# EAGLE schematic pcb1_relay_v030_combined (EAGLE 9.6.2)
Minor corrections.

## Sheet 1 of 3: Signal Generator
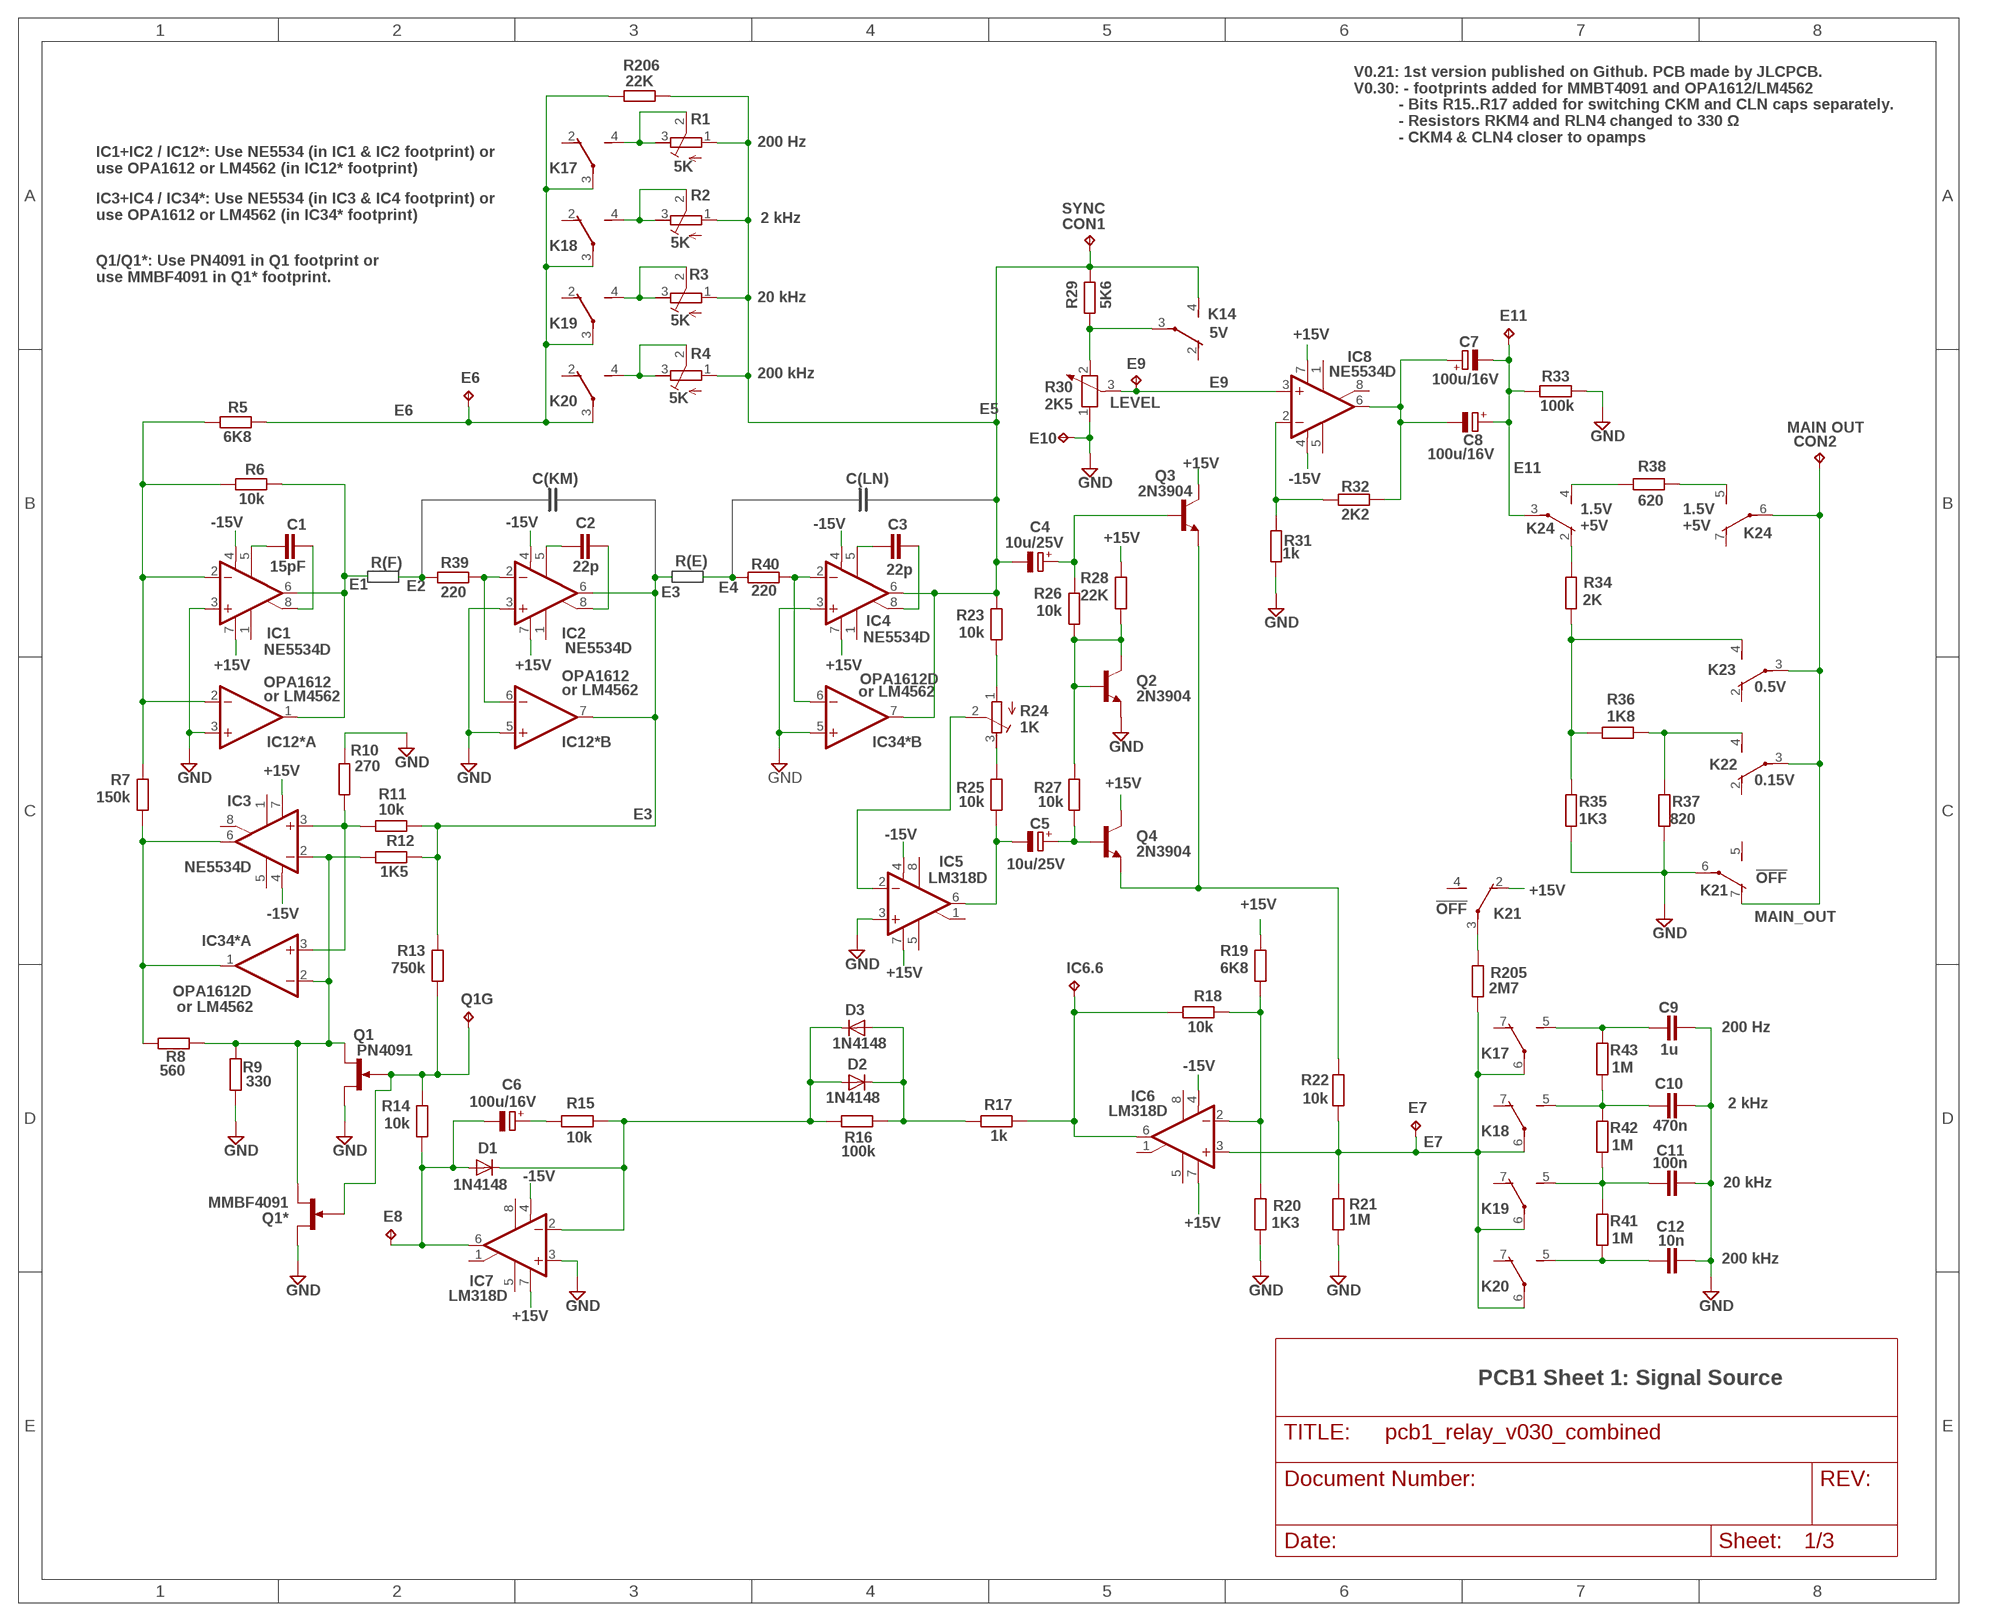
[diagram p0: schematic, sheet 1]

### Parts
C1  15pF  C-EU075-042X103  [C075-042X103]
C2  22p  C-EU075-042X103  [C075-042X103]
C3  22p  C-EU075-042X103  [C075-042X103]
C4  10u/25V  CPOL-EUUD-4X5,8  [UD-4X5,8_NICHICON]
C5  10u/25V  CPOL-EUUD-4X5,8  [UD-4X5,8_NICHICON]
C6  100u/16V  CPOL-EUUD-6,3X8,8  [UD-6,3X5,8_NICHICON]
C7  100u/16V  CPOL-EUUD-6,3X8,8  [UD-6,3X5,8_NICHICON]
C8  100u/16V  CPOL-EUUD-6,3X8,8  [UD-6,3X5,8_NICHICON]
C9  1u  C-EU150-072X183  [C150-072X183]
C10  470n  C-EU102-064X133  [C102-064X133]
C11  100n  C-EU075-063X106  [C075-063X106]
C12  10n  C-EU050-045X075  [C050-045X075]
CON1  MAIN_OUT  TPPAD1-13Y  [P1-13Y]
CON2  MAIN_OUT  TPPAD1-13Y  [P1-13Y]
D1  1N4148  D-SOD-80  [SOD80]
D2  1N4148  D-SOD-80  [SOD80]
D3  1N4148  D-SOD-80  [SOD80]
E6  TPPAD1-13Y  [P1-13Y]
E7  TPPAD1-13Y  [P1-13Y]
E8  TPPAD1-13Y  [P1-13Y]
E9  TPPAD1-13Y  [P1-13Y]
E10  MAIN_OUT  TPPAD1-13Y  [P1-13Y]
E11  TPPAD1-13Y  [P1-13Y]
IC1  NE5534D  NE5534AD  [SO08]
IC2  NE5534D  NE5534AD  [SO08]
IC3  NE5534D  NE5534AD  [SO08]
IC4  NE5534D  NE5534AD  [SO08]
IC5  LM318D  [SO08]
IC6  LM318D  [SO08]
IC6.6  TPPAD1-13Y  [P1-13Y]
IC7  LM318D  [SO08]
IC8  NE5534D  NE5534AD  [SO08]
IC12*  OPA1612  OPA1013D  [SO08]
IC34*  OPA1612D  OPA1013D  [SO08]
K14  G6K-2F-Y  [G6K-2F-Y]
K17  G6K-2F-Y  [G6K-2F-Y]
K18  G6K-2F-Y  [G6K-2F-Y]
K19  G6K-2F-Y  [G6K-2F-Y]
K20  G6K-2F-Y  [G6K-2F-Y]
K21  G6K-2F-Y  [G6K-2F-Y]
K22  G6K-2F-Y  [G6K-2F-Y]
K23  G6K-2F-Y  [G6K-2F-Y]
K24  G6K-2F-Y  [G6K-2F-Y]
Q1  PN4091  2N5638  [TO92G]
Q1*  MMBF4091  MMBFJ3  [SOT23]
Q1G  TPPAD1-13Y  [P1-13Y]
Q2  2N3904  [TO92]
Q3  2N3904  [TO92]
Q4  2N3904  [TO92]
R1  5K  R-TRIMM3296W  [RTRIM3296W]
R2  5K  R-TRIMM3296W  [RTRIM3296W]
R3  5K  R-TRIMM3296W  [RTRIM3296W]
R4  5K  R-TRIMM3296W  [RTRIM3296W]
R5  6K8  R-EU_R1206  [R1206]
R6  10k  R-EU_R1206  [R1206]
R7  150k  R-EU_R1206  [R1206]
R8  560  R-EU_R1206  [R1206]
R9  330  R-EU_R1206  [R1206]
R10  270  R-EU_R1206  [R1206]
R11  10k  R-EU_R1206  [R1206]
R12  1K5  R-EU_R1206  [R1206]
R13  750k  R-EU_R1206  [R1206]
R14  10k  R-EU_R1206  [R1206]
R15  10k  R-EU_R1206  [R1206]
R16  100k  R-EU_R1206  [R1206]
R17  1k  R-EU_R1206  [R1206]
R18  10k  R-EU_R1206  [R1206]
R19  6K8  R-EU_R1206  [R1206]
R20  1K3  R-EU_R1206  [R1206]
R21  1M  R-EU_R1206  [R1206]
R22  10k  R-EU_R1206  [R1206]
R23  10k  R-EU_R1206  [R1206]
R24  1K  R-TRIMM3296W  [RTRIM3296W]
R25  10k  R-EU_R1206  [R1206]
R26  10k  R-EU_R1206  [R1206]
R27  10k  R-EU_R1206  [R1206]
R28  22K  R-EU_R1206  [R1206]
R29  5K6  R-EU_R1206  [R1206]
R30  2K5  POTENTIOMETER_PT-10S  [PT-10S]
R31  1k  R-EU_R1206  [R1206]
R32  2K2  R-EU_R1206  [R1206]
R33  100k  R-EU_R1206  [R1206]
R34  2K  R-EU_R1206  [R1206]
R35  1K3  R-EU_R1206  [R1206]
R36  1K8  R-EU_R1206  [R1206]
R37  820  R-EU_R1206  [R1206]
R38  620  R-EU_R1206  [R1206]
R39  220  R-EU_R1206  [R1206]
R40  220  R-EU_R1206  [R1206]
R41  1M  R-EU_R1206  [R1206]
R42  1M  R-EU_R1206  [R1206]
R43  1M  R-EU_R1206  [R1206]
R205  2M7  R-EU_R1206  [R1206]
R206  22K  R-EU_R1206  [R1206]

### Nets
+15V: IC1.7(V+) IC2.7(V+) IC3.7(V+) IC4.7(V+) IC5.7(V+) IC6.7(V+) IC7.7(V+) IC8.7(V+) K21.2(2:O) Q3.1(C) Q4.1(C) R19.2 R28.2 ; also sheet 3
-15V: IC1.4(V-) IC2.4(V-) IC3.4(V-) IC4.4(V-) IC5.4(V-) IC6.4(V-) IC7.4(V-) IC8.4(V-) ; also sheet 3
E1: IC1.6(OUT) IC12*.1(A:OUT) R6.2 ; also sheet 2
E2: R39.1 ; also sheet 2
E3: IC2.6(OUT) IC12*.7(B:OUT) R11.2 R12.2 R13.2 ; also sheet 2
E4: R40.1 ; also sheet 2
E5: C4.- CON1.TP IC4.6(OUT) IC34*.7(B:OUT) K14.4(2:S) R1.1(A) R2.1(A) R3.1(A) R4.1(A) R23.2 R29.2 R206.2 ; also sheet 2
E6: E6.TP K17.3(2:P) K18.3(2:P) K19.3(2:P) K20.3(2:P) R5.2 R206.1
E7: E7.TP IC6.3(+IN) K17.6(3:P) K18.6(3:P) K19.6(3:P) K20.6(3:P) R21.1 R22.2 R205.2
E8: C6.- D1.2(A) E8.TP IC7.6(OUT) R14.1
E9: E9.TP IC8.3(+IN) R30.3
E11: C7.- C8.+ E11.TP K24.3(2:P) R33.1
GND: C9.2 C10.2 C11.2 C12.2 E10.TP IC1.3(+IN) IC2.3(+IN) IC4.3(+IN) IC5.3(+IN) IC7.3(+IN) IC12*.3(A:+IN) IC12*.5(B:+IN) IC34*.5(B:+IN) K21.6(3:P) Q1*.1(D) Q1.S Q2.3(E) R9.1 R10.2 R20.2 R21.2 R30.1 R31.1 R33.2 R35.1 R37.1 ; also sheet 2,3
IC1P5: C1.2 IC1.5(CMP)
IC2P5: C2.2 IC2.5(CMP)
IC4P5: C3.2 IC4.5(CMP)
IC6.6: IC6.6(OUT) IC6.6.TP R17.2 R18.1
MAIN_OUT: CON2.TP K21.7(3:O) K22.3(2:P) K23.3(2:P) K24.6(3:P) ; also sheet 2
N$4: C1.1 IC1.8(ON/CMP)
N$6: K20.4(2:S) R4.2(S) R4.3(E)
N$9: IC1.2(-IN) IC12*.2(A:-IN) R5.1 R6.1 R7.2
N$11: IC2.2(-IN) IC12*.6(B:-IN) R39.2
N$14: C2.1 IC2.8(ON/CMP)
N$15: IC3.3(+IN) IC34*.3(A:+IN) R10.1 R11.1
N$16: IC3.6(OUT) IC34*.1(A:OUT) R7.1 R8.1
N$17: Q1*.3(G) Q1.G Q1G.TP R13.1 R14.2
N$18: IC3.2(-IN) IC34*.2(A:-IN) Q1*.2(S) Q1.D R8.2 R9.2 R12.1
N$20: IC4.2(-IN) IC34*.6(B:-IN) R40.2
N$23: C6.+ R15.1
N$24: D2.1(C) D3.2(A) R16.2 R17.1
N$25: D1.1(C) D2.2(A) D3.1(C) IC7.2(-IN) R15.2 R16.1
N$27: IC6.2(-IN) R18.2 R19.1 R20.1
N$30: Q3.3(E) Q4.3(E) R22.1
N$31: C5.+ Q4.2(B) R27.1
N$33: C5.- IC5.6(OUT) R25.1
N$34: Q2.1(C) Q2.2(B) R26.1 R27.2 R28.1
N$35: K23.4(2:S) R34.2 R35.2 R36.2
N$71: C3.1 IC4.8(ON/CMP)
N$76: C4.+ Q3.2(B) R26.2
N$83: C9.1 K17.5(3:S) R43.2
N$84: K19.4(2:S) R3.2(S) R3.3(E)
N$85: K17.4(2:S) R1.2(S) R1.3(E)
N$86: K18.4(2:S) R2.2(S) R2.3(E)
N$87: C10.1 K18.5(3:S) R42.2 R43.1
N$88: C11.1 K19.5(3:S) R41.2 R42.1
N$89: C12.1 K20.5(3:S) R41.1
N$96: K21.3(2:P) R205.1
N$97: R23.1 R24.1(A)
N$98: K22.4(2:S) R36.1 R37.2
N$99: K24.4(2:S) R38.1
N$100: K24.5(3:S) R38.2
N$101: K24.2(2:O) R34.1
N$102: K14.3(2:P) R29.1 R30.2
N$117: R24.3(E) R25.2
N$118: IC5.2(-IN) R24.2(S)
N$120: C7.+ C8.- IC8.6(OUT) R32.2
N$121: IC8.2(-IN) R31.2 R32.1
Unconnected: IC1.1(ON) IC2.1(ON) IC3.1(ON) IC3.5(CMP) IC3.8(ON/CMP) IC4.1(ON) IC5.1(ON/CMP) IC5.5(ON) IC5.8(CMP) IC6.1(ON/CMP) IC6.5(ON) IC6.8(CMP) IC7.1(ON/CMP) IC7.5(ON) IC7.8(CMP) IC8.1(ON) IC8.5(CMP) IC8.8(ON/CMP) K14.2(2:O) K17.2(2:O) K17.7(3:O) K18.2(2:O) K18.7(3:O) K19.2(2:O) K19.7(3:O) K20.2(2:O) K20.7(3:O) K21.4(2:S) K21.5(3:S) K22.2(2:O) K23.2(2:O) K24.7(3:O)

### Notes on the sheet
- V0.21: 1st version published on Github. PCB made by JLCPCB.
  V0.30: - footprints added for MMBT4091 and OPA1612/LM4562
            - Bits R15..R17 added for switching CKM and CLN caps separately.
            - Resistors RKM4 and RLN4 changed to 330 Ω
            - CKM4 & CLN4 closer to opamps
- 200 Hz
- IC1+IC2 / IC12*: Use NE5534 (in IC1 & IC2 footprint) or
  use OPA1612 or LM4562 (in IC12* footprint)
- SYNC
- IC3+IC4 / IC34*: Use NE5534 (in IC3 & IC4 footprint) or
  use OPA1612 or LM4562 (in IC34* footprint)
- 2 kHz
- Q1/Q1*: Use PN4091 in Q1 footprint or
  use MMBF4091 in Q1* footprint.
- 20 kHz
- 5V
- 200 kHz
- LEVEL
- MAIN OUT
- C(KM) | C(LN)
- 1.5V
  +5V
- 1.5V
  +5V
- R(F) | R(E)
- or LM4562 | 0.5V
- or LM4562
- or LM4562
- 0.15V
- !OFF
- !OFF
- or LM4562
- 200 Hz
- 2 kHz
- 20 kHz
- 200 kHz
- PCB1 Sheet 1: Signal Source

## Sheet 2 of 3: Relays + Digital Logic
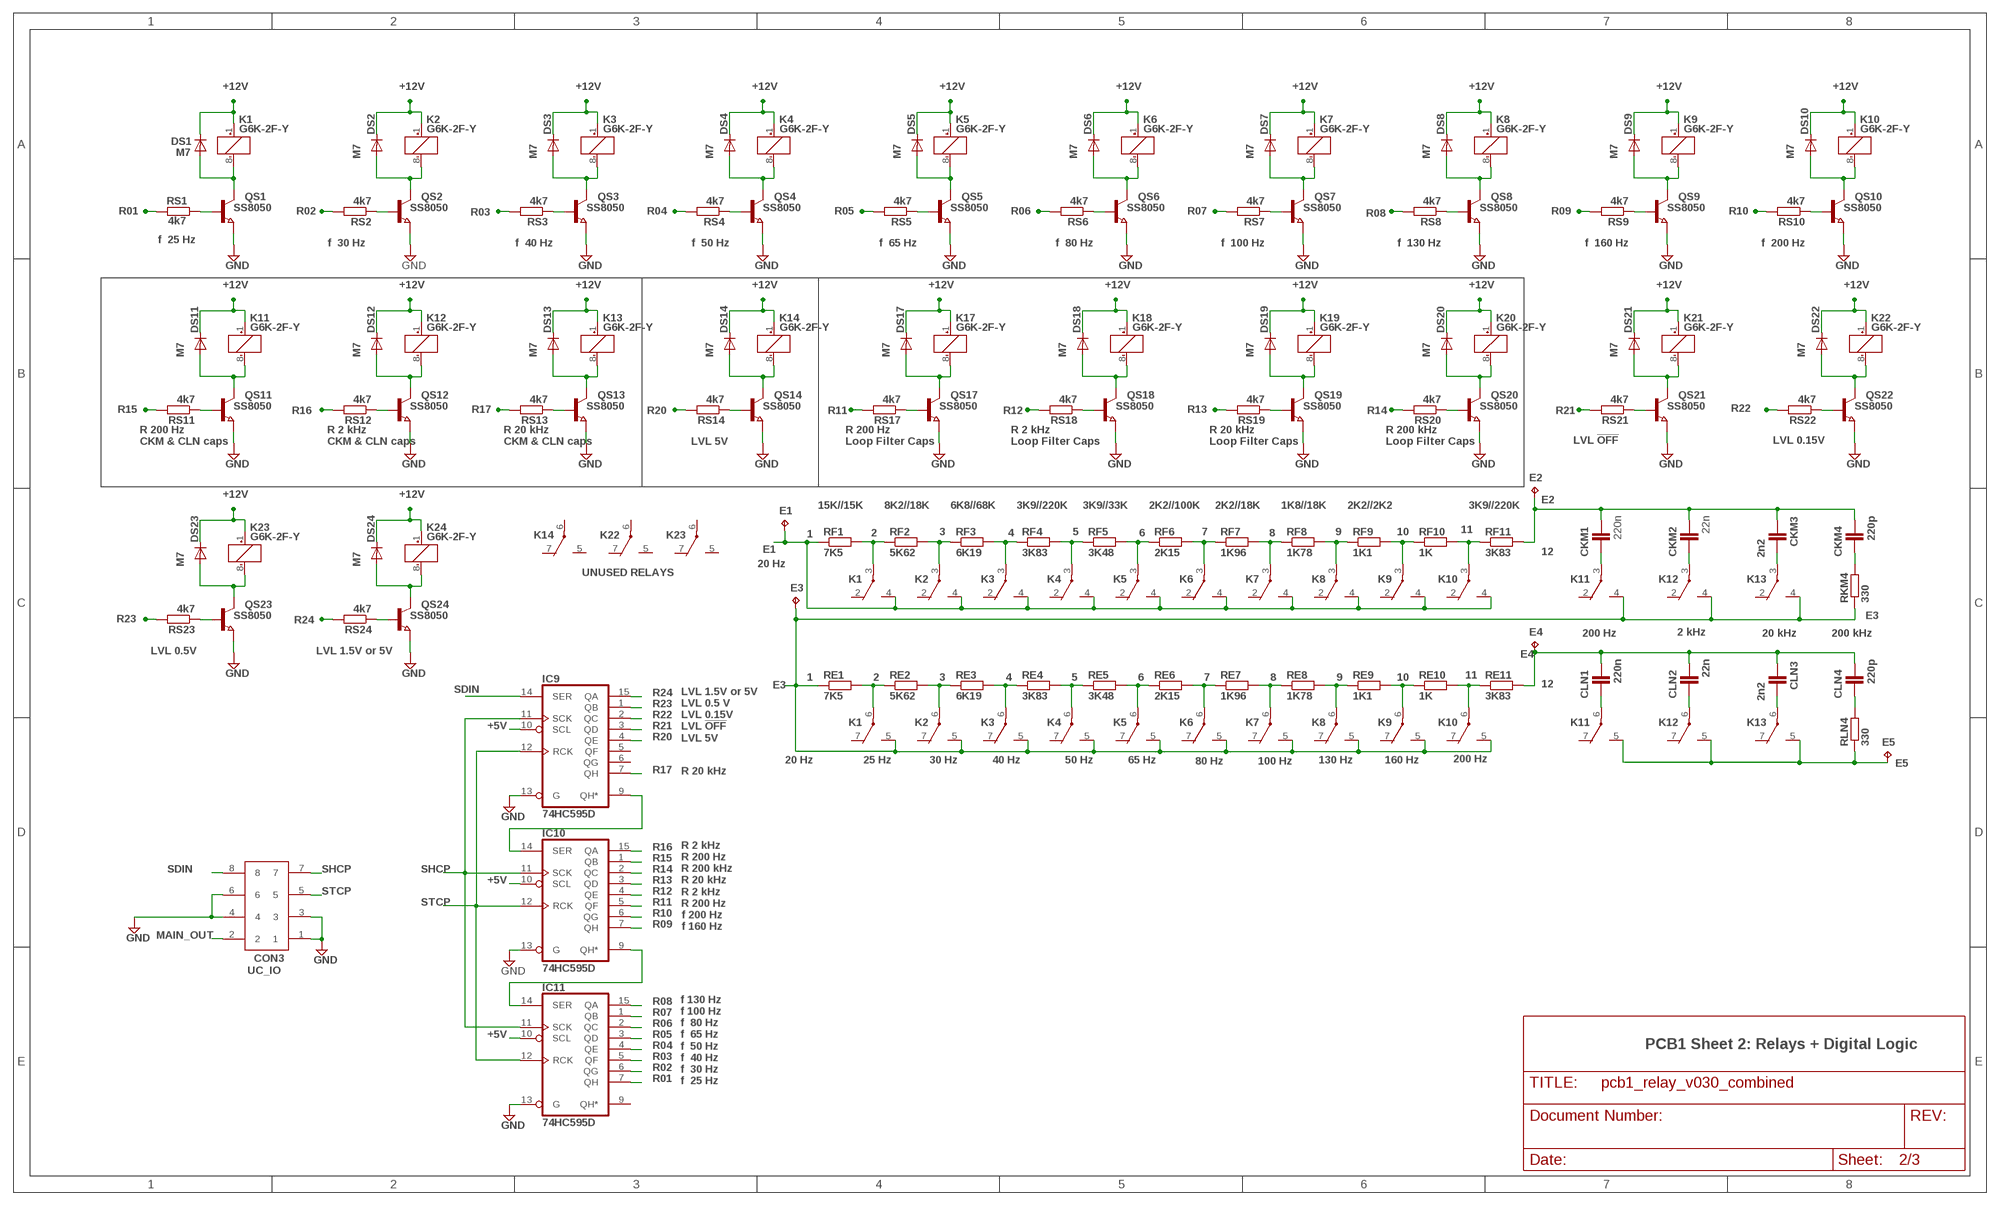
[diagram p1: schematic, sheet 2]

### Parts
CKM1  220n  C-EU075-052X106  [C075-052X106]
CKM2  22n  C-EU050-045X075  [C050-045X075]
CKM3  2n2  C-EU075-052X106  [C075-052X106]
CKM4  220p  C-EU075-052X106  [C075-052X106]
CLN1  220n  C-EU075-052X106  [C075-052X106]
CLN2  22n  C-EU050-045X075  [C050-045X075]
CLN3  2n2  C-EU075-052X106  [C075-052X106]
CLN4  220p  C-EU075-052X106  [C075-052X106]
CON3  UC_IO  61200821621  [61200821621]
DS1  M7  DIODE-DO214AC  [DO214AC]
DS2  M7  DIODE-DO214AC  [DO214AC]
DS3  M7  DIODE-DO214AC  [DO214AC]
DS4  M7  DIODE-DO214AC  [DO214AC]
DS5  M7  DIODE-DO214AC  [DO214AC]
DS6  M7  DIODE-DO214AC  [DO214AC]
DS7  M7  DIODE-DO214AC  [DO214AC]
DS8  M7  DIODE-DO214AC  [DO214AC]
DS9  M7  DIODE-DO214AC  [DO214AC]
DS10  M7  DIODE-DO214AC  [DO214AC]
DS11  M7  DIODE-DO214AC  [DO214AC]
DS12  M7  DIODE-DO214AC  [DO214AC]
DS13  M7  DIODE-DO214AC  [DO214AC]
DS14  M7  DIODE-DO214AC  [DO214AC]
DS17  M7  DIODE-DO214AC  [DO214AC]
DS18  M7  DIODE-DO214AC  [DO214AC]
DS19  M7  DIODE-DO214AC  [DO214AC]
DS20  M7  DIODE-DO214AC  [DO214AC]
DS21  M7  DIODE-DO214AC  [DO214AC]
DS22  M7  DIODE-DO214AC  [DO214AC]
DS23  M7  DIODE-DO214AC  [DO214AC]
DS24  M7  DIODE-DO214AC  [DO214AC]
E1  TPPAD1-13Y  [P1-13Y]
E2  TPPAD1-13Y  [P1-13Y]
E3  TPPAD1-13Y  [P1-13Y]
E4  TPPAD1-13Y  [P1-13Y]
E5  TPPAD1-13Y  [P1-13Y]
IC9  74HC595D  [SO16]
IC10  74HC595D  [SO16]
IC11  74HC595D  [SO16]
K1  G6K-2F-Y  [G6K-2F-Y]
K2  G6K-2F-Y  [G6K-2F-Y]
K3  G6K-2F-Y  [G6K-2F-Y]
K4  G6K-2F-Y  [G6K-2F-Y]
K5  G6K-2F-Y  [G6K-2F-Y]
K6  G6K-2F-Y  [G6K-2F-Y]
K7  G6K-2F-Y  [G6K-2F-Y]
K8  G6K-2F-Y  [G6K-2F-Y]
K9  G6K-2F-Y  [G6K-2F-Y]
K10  G6K-2F-Y  [G6K-2F-Y]
K11  G6K-2F-Y  [G6K-2F-Y]
K12  G6K-2F-Y  [G6K-2F-Y]
K13  G6K-2F-Y  [G6K-2F-Y]
QS1  SS8050  NPN-TRANSISTOR_SOT23  [SOT23]
QS2  SS8050  NPN-TRANSISTOR_SOT23  [SOT23]
QS3  SS8050  NPN-TRANSISTOR_SOT23  [SOT23]
QS4  SS8050  NPN-TRANSISTOR_SOT23  [SOT23]
QS5  SS8050  NPN-TRANSISTOR_SOT23  [SOT23]
QS6  SS8050  NPN-TRANSISTOR_SOT23  [SOT23]
QS7  SS8050  NPN-TRANSISTOR_SOT23  [SOT23]
QS8  SS8050  NPN-TRANSISTOR_SOT23  [SOT23]
QS9  SS8050  NPN-TRANSISTOR_SOT23  [SOT23]
QS10  SS8050  NPN-TRANSISTOR_SOT23  [SOT23]
QS11  SS8050  NPN-TRANSISTOR_SOT23  [SOT23]
QS12  SS8050  NPN-TRANSISTOR_SOT23  [SOT23]
QS13  SS8050  NPN-TRANSISTOR_SOT23  [SOT23]
QS14  SS8050  NPN-TRANSISTOR_SOT23  [SOT23]
QS17  SS8050  NPN-TRANSISTOR_SOT23  [SOT23]
QS18  SS8050  NPN-TRANSISTOR_SOT23  [SOT23]
QS19  SS8050  NPN-TRANSISTOR_SOT23  [SOT23]
QS20  SS8050  NPN-TRANSISTOR_SOT23  [SOT23]
QS21  SS8050  NPN-TRANSISTOR_SOT23  [SOT23]
QS22  SS8050  NPN-TRANSISTOR_SOT23  [SOT23]
QS23  SS8050  NPN-TRANSISTOR_SOT23  [SOT23]
QS24  SS8050  NPN-TRANSISTOR_SOT23  [SOT23]
RE1  7K5  R-EU_R1206  [R1206]
RE2  5K62  R-EU_R1206  [R1206]
RE3  6K19  R-EU_R1206  [R1206]
RE4  3K83  R-EU_R1206  [R1206]
RE5  3K48  R-EU_R1206  [R1206]
RE6  2K15  R-EU_R1206  [R1206]
RE7  1K96  R-EU_R1206  [R1206]
RE8  1K78  R-EU_R1206  [R1206]
RE9  1K1  R-EU_R1206  [R1206]
RE10  1K  R-EU_R1206  [R1206]
RE11  3K83  R-EU_R1206  [R1206]
RF1  7K5  R-EU_R1206  [R1206]
RF2  5K62  R-EU_R1206  [R1206]
RF3  6K19  R-EU_R1206  [R1206]
RF4  3K83  R-EU_R1206  [R1206]
RF5  3K48  R-EU_R1206  [R1206]
RF6  2K15  R-EU_R1206  [R1206]
RF7  1K96  R-EU_R1206  [R1206]
RF8  1K78  R-EU_R1206  [R1206]
RF9  1K1  R-EU_R1206  [R1206]
RF10  1K  R-EU_R1206  [R1206]
RF11  3K83  R-EU_R1206  [R1206]
RKM4  330  R-EU_R1206  [R1206]
RLN4  330  R-EU_R1206  [R1206]
RS1  4k7  R-EU_M1206  [M1206]
RS2  4k7  R-EU_M1206  [M1206]
RS3  4k7  R-EU_M1206  [M1206]
RS4  4k7  R-EU_M1206  [M1206]
RS5  4k7  R-EU_M1206  [M1206]
RS6  4k7  R-EU_M1206  [M1206]
RS7  4k7  R-EU_M1206  [M1206]
RS8  4k7  R-EU_M1206  [M1206]
RS9  4k7  R-EU_M1206  [M1206]
RS10  4k7  R-EU_M1206  [M1206]
RS11  4k7  R-EU_M1206  [M1206]
RS12  4k7  R-EU_M1206  [M1206]
RS13  4k7  R-EU_M1206  [M1206]
RS14  4k7  R-EU_M1206  [M1206]
RS17  4k7  R-EU_M1206  [M1206]
RS18  4k7  R-EU_M1206  [M1206]
RS19  4k7  R-EU_M1206  [M1206]
RS20  4k7  R-EU_M1206  [M1206]
RS21  4k7  R-EU_M1206  [M1206]
RS22  4k7  R-EU_M1206  [M1206]
RS23  4k7  R-EU_M1206  [M1206]
RS24  4k7  R-EU_M1206  [M1206]

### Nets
+5V: IC9.10(SCL) IC10.10(SCL) IC11.10(SCL) ; also sheet 3
+12V: DS1.C DS2.C DS3.C DS4.C DS5.C DS6.C DS7.C DS8.C DS9.C DS10.C DS11.C DS12.C DS13.C DS14.C DS17.C DS18.C DS19.C DS20.C DS21.C DS22.C DS23.C DS24.C K1.1(1:+) K2.1(1:+) K3.1(1:+) K4.1(1:+) K5.1(1:+) K6.1(1:+) K7.1(1:+) K8.1(1:+) K9.1(1:+) K10.1(1:+) K11.1(1:+) K12.1(1:+) K13.1(1:+) K14.1(1:+) K17.1(1:+) K18.1(1:+) K19.1(1:+) K20.1(1:+) K21.1(1:+) K22.1(1:+) K23.1(1:+) K24.1(1:+) ; also sheet 3
E1: E1.TP K1.4(2:S) K2.4(2:S) K3.4(2:S) K4.4(2:S) K5.4(2:S) K6.4(2:S) K7.4(2:S) K8.4(2:S) K9.4(2:S) K10.4(2:S) RF1.1 ; also sheet 1
E2: CKM1.2 CKM2.2 CKM3.1 CKM4.2 E2.TP RF11.2 ; also sheet 1
E3: E3.TP K1.5(3:S) K2.5(3:S) K3.5(3:S) K4.5(3:S) K5.5(3:S) K6.5(3:S) K7.5(3:S) K8.5(3:S) K9.5(3:S) K10.5(3:S) K11.4(2:S) K12.4(2:S) K13.4(2:S) RE1.1 RKM4.1 ; also sheet 1
E4: CLN1.2 CLN2.2 CLN3.1 CLN4.2 E4.TP RE11.2 ; also sheet 1
E5: E5.TP K11.5(3:S) K12.5(3:S) K13.5(3:S) RLN4.1 ; also sheet 1
GND: CON3.1 CON3.3 CON3.4 CON3.6 IC9.13(G) IC10.13(G) IC11.13(G) QS1.2(E) QS2.2(E) QS3.2(E) QS4.2(E) QS5.2(E) QS6.2(E) QS7.2(E) QS8.2(E) QS9.2(E) QS10.2(E) QS11.2(E) QS12.2(E) QS13.2(E) QS14.2(E) QS17.2(E) QS18.2(E) QS19.2(E) QS20.2(E) QS21.2(E) QS22.2(E) QS23.2(E) QS24.2(E) ; also sheet 1,3
MAIN_OUT: CON3.2 ; also sheet 1
N$1: CKM4.1 RKM4.2
N$2: CLN4.1 RLN4.2
N$3: K1.3(2:P) RF1.2 RF2.1
N$5: K2.3(2:P) RF2.2 RF3.1
N$8: K3.3(2:P) RF3.2 RF4.1
N$13: K4.3(2:P) RF4.2 RF5.1
N$21: QS11.1(B) RS11.1
N$28: K5.3(2:P) RF5.2 RF6.1
N$32: QS24.1(B) RS24.1
N$36: K6.3(2:P) RF6.2 RF7.1
N$37: K7.3(2:P) RF7.2 RF8.1
N$38: K8.3(2:P) RF8.2 RF9.1
N$39: K9.3(2:P) RF9.2 RF10.1
N$40: K10.3(2:P) RF10.2 RF11.1
N$41: K1.6(3:P) RE1.2 RE2.1
N$42: K2.6(3:P) RE2.2 RE3.1
N$43: K3.6(3:P) RE3.2 RE4.1
N$44: K4.6(3:P) RE4.2 RE5.1
N$45: K5.6(3:P) RE5.2 RE6.1
N$46: K6.6(3:P) RE6.2 RE7.1
N$47: K7.6(3:P) RE7.2 RE8.1
N$48: K8.6(3:P) RE8.2 RE9.1
N$49: K9.6(3:P) RE9.2 RE10.1
N$50: K10.6(3:P) RE10.2 RE11.1
N$51: QS1.1(B) RS1.1
N$52: DS1.A K1.8(1:-) QS1.3(C)
N$53: QS2.1(B) RS2.1
N$54: DS2.A K2.8(1:-) QS2.3(C)
N$55: QS3.1(B) RS3.1
N$56: DS3.A K3.8(1:-) QS3.3(C)
N$57: QS4.1(B) RS4.1
N$58: DS4.A K4.8(1:-) QS4.3(C)
N$59: QS5.1(B) RS5.1
N$60: DS5.A K5.8(1:-) QS5.3(C)
N$61: QS6.1(B) RS6.1
N$62: DS6.A K6.8(1:-) QS6.3(C)
N$63: QS7.1(B) RS7.1
N$64: DS7.A K7.8(1:-) QS7.3(C)
N$65: QS8.1(B) RS8.1
N$66: DS8.A K8.8(1:-) QS8.3(C)
N$67: QS9.1(B) RS9.1
N$68: DS9.A K9.8(1:-) QS9.3(C)
N$69: QS10.1(B) RS10.1
N$70: DS10.A K10.8(1:-) QS10.3(C)
N$72: CKM1.1 K11.3(2:P)
N$73: CKM2.1 K12.3(2:P)
N$74: CKM3.2 K13.3(2:P)
N$75: DS11.A K11.8(1:-) QS11.3(C)
N$77: QS12.1(B) RS12.1
N$78: DS12.A K12.8(1:-) QS12.3(C)
N$79: QS13.1(B) RS13.1
N$80: DS13.A K13.8(1:-) QS13.3(C)
N$81: QS14.1(B) RS14.1
N$82: DS14.A K14.8(1:-) QS14.3(C)
N$90: QS18.1(B) RS18.1
N$91: DS18.A K18.8(1:-) QS18.3(C)
N$92: QS19.1(B) RS19.1
N$93: DS19.A K19.8(1:-) QS19.3(C)
N$94: QS20.1(B) RS20.1
N$95: DS20.A K20.8(1:-) QS20.3(C)
N$103: QS21.1(B) RS21.1
N$104: DS21.A K21.8(1:-) QS21.3(C)
N$105: QS22.1(B) RS22.1
N$106: DS22.A K22.8(1:-) QS22.3(C)
N$107: QS23.1(B) RS23.1
N$108: DS23.A K23.8(1:-) QS23.3(C)
N$109: DS24.A K24.8(1:-) QS24.3(C)
N$110: QS17.1(B) RS17.1
N$111: DS17.A K17.8(1:-) QS17.3(C)
N$112: IC9.9(QH*) IC10.14(SER)
N$113: IC10.9(QH*) IC11.14(SER)
N$114: CLN1.1 K11.6(3:P)
N$115: CLN2.1 K12.6(3:P)
N$116: CLN3.2 K13.6(3:P)
R01: IC11.7(QH) RS1.2
R02: IC11.6(QG) RS2.2
R03: IC11.5(QF) RS3.2
R04: IC11.4(QE) RS4.2
R05: IC11.3(QD) RS5.2
R06: IC11.2(QC) RS6.2
R07: IC11.1(QB) RS7.2
R08: IC11.15(QA) RS8.2
R09: IC10.7(QH) RS9.2
R10: IC10.6(QG) RS10.2
R11: IC10.5(QF) RS17.2
R12: IC10.4(QE) RS18.2
R13: IC10.3(QD) RS19.2
R14: IC10.2(QC) RS20.2
R15: IC10.1(QB) RS11.2
R16: IC10.15(QA) RS12.2
R17: IC9.7(QH) RS13.2
R20: IC9.4(QE) RS14.2
R21: IC9.3(QD) RS21.2
R22: IC9.2(QC) RS22.2
R23: IC9.1(QB) RS23.2
R24: IC9.15(QA) RS24.2
SDIN: CON3.8 IC9.14(SER)
SHCP: CON3.7 IC9.11(SCK) IC10.11(SCK) IC11.11(SCK)
STCP: CON3.5 IC9.12(RCK) IC10.12(RCK) IC11.12(RCK)
Unconnected: IC9.5(QF) IC9.6(QG) IC11.9(QH*) K1.2(2:O) K1.7(3:O) K2.2(2:O) K2.7(3:O) K3.2(2:O) K3.7(3:O) K4.2(2:O) K4.7(3:O) K5.2(2:O) K5.7(3:O) K6.2(2:O) K6.7(3:O) K7.2(2:O) K7.7(3:O) K8.2(2:O) K8.7(3:O) K9.2(2:O) K9.7(3:O) K10.2(2:O) K10.7(3:O) K11.2(2:O) K11.7(3:O) K12.2(2:O) K12.7(3:O) K13.2(2:O) K13.7(3:O) K14.5(3:S) K14.6(3:P) K14.7(3:O) K22.5(3:S) K22.6(3:P) K22.7(3:O) K23.5(3:S) K23.6(3:P) K23.7(3:O)

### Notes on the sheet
- f  25 Hz
- f  30 Hz | f  40 Hz | f  50 Hz | f  65 Hz | f  80 Hz | f  100 Hz | f  130 Hz | f  160 Hz | f  200 Hz
- LVL !OFF | LVL 0.15V
- R 200 Hz
  CKM & CLN caps
- R 2 kHz
  CKM & CLN caps
- R 20 kHz
  CKM & CLN caps
- LVL 5V
- R 200 Hz
  Loop Filter Caps
- R 2 kHz
  Loop Filter Caps
- R 20 kHz
  Loop Filter Caps
- R 200 kHz
  Loop Filter Caps
- 15K//15K | 8K2//18K | 6K8//68K | 3K9//220K | 3K9//33K | 2K2//100K | 2K2//18K | 1K8//18K | 2K2//2K2 | 3K9//220K
- 3 | 5 | 7 | 9 | 10 | 11
- 1 | 2 | 4 | 6 | 8
- 12
- 20 Hz
- UNUSED RELAYS
- 200 Hz | 2 kHz | 20 kHz | 200 kHz
- LVL 0.5V | LVL 1.5V or 5V
- 1 | 2 | 3 | 4 | 5 | 6 | 7 | 8 | 9 | 10 | 11
- 12
- LVL 1.5V or 5V
  LVL 0.5 V
  LVL 0.15V
  LVL !OFF
  LVL 5V
- 20 Hz | 25 Hz | 30 Hz | 40 Hz | 50 Hz | 65 Hz | 80 Hz | 100 Hz | 130 Hz | 160 Hz | 200 Hz
- R 20 kHz
- R 2 kHz
  R 200 Hz
  R 200 kHz
  R 20 kHz
  R 2 kHz
  R 200 Hz
  f 200 Hz
  f 160 Hz
- PCB1 Sheet 2: Relays + Digital Logic
- f 130 Hz
  f 100 Hz
  f  80 Hz
  f  65 Hz
  f  50 Hz
  f  40 Hz
  f  30 Hz
  f  25 Hz

## Sheet 3 of 3: Power Supply
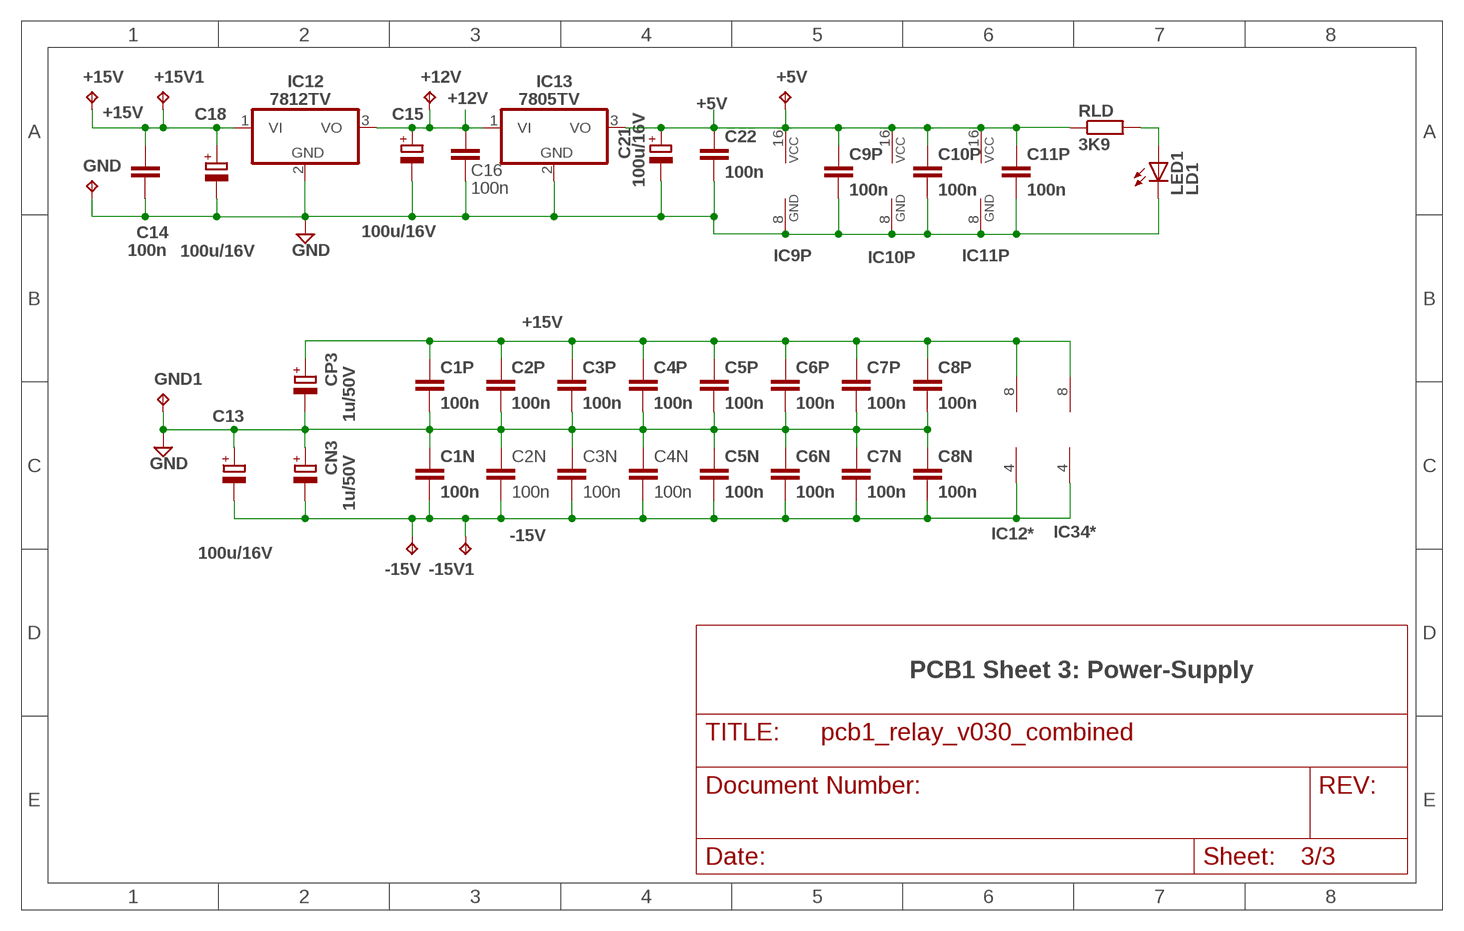
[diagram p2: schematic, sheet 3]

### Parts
+5V  TPPAD1-13Y  [P1-13Y]
+12V  TPPAD1-13Y  [P1-13Y]
+15V  TPPAD1-13Y  [P1-13Y]
+15V1  TPPAD1-13Y  [P1-13Y]
-15V  TPPAD1-13Y  [P1-13Y]
-15V1  TPPAD1-13Y  [P1-13Y]
C1N  100n  C-EUC1206  [C1206]
C1P  100n  C-EUC1206  [C1206]
C2N  100n  C-EUC1206  [C1206]
C2P  100n  C-EUC1206  [C1206]
C3N  100n  C-EUC1206  [C1206]
C3P  100n  C-EUC1206  [C1206]
C4N  100n  C-EUC1206  [C1206]
C4P  100n  C-EUC1206  [C1206]
C5N  100n  C-EUC1206  [C1206]
C5P  100n  C-EUC1206  [C1206]
C6N  100n  C-EUC1206  [C1206]
C6P  100n  C-EUC1206  [C1206]
C7N  100n  C-EUC1206  [C1206]
C7P  100n  C-EUC1206  [C1206]
C8N  100n  C-EUC1206  [C1206]
C8P  100n  C-EUC1206  [C1206]
C9P  100n  C-EUC1206  [C1206]
C10P  100n  C-EUC1206  [C1206]
C11P  100n  C-EUC1206  [C1206]
C13  100u/16V  CPOL-EUUD-6,3X8,8  [UD-6,3X5,8_NICHICON]
C14  100n  C-EUC1206  [C1206]
C15  100u/16V  CPOL-EUUD-6,3X8,8  [UD-6,3X5,8_NICHICON]
C16  100n  C-EUC1206  [C1206]
C18  100u/16V  CPOL-EUUD-6,3X8,8  [UD-6,3X5,8_NICHICON]
C21  100u/16V  CPOL-EUUD-6,3X8,8  [UD-6,3X5,8_NICHICON]
C22  100n  C-EUC1206  [C1206]
CN3  1u/50V  CPOL-EUUD-4X5,8  [UD-4X5,8_NICHICON]
CP3  1u/50V  CPOL-EUUD-4X5,8  [UD-4X5,8_NICHICON]
GND  TPPAD1-13Y  [P1-13Y]
GND1  TPPAD1-13Y  [P1-13Y]
IC12  7812TV  [TO220V]
IC13  7805TV  [TO220V]
LED1  LD1  LEDCHIPLED_1206  [CHIPLED_1206]
RLD  3K9  R-EU_R1206  [R1206]

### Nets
+5V: +5V.TP C9P.1 C10P.1 C11P.1 C21.+ C22.1 IC9.16(VCC) IC10.16(VCC) IC11.16(VCC) IC13.3(VO) RLD.1 ; also sheet 2
+12V: +12V.TP C15.+ C16.1 IC12.3(VO) IC13.1(VI) ; also sheet 2
+15V: +15V1.TP +15V.TP C1P.1 C2P.1 C3P.1 C4P.1 C5P.1 C6P.1 C7P.1 C8P.1 C14.1 C18.+ CP3.+ IC12*.8(P:V+) IC12.1(VI) IC34*.8(P:V+) ; also sheet 1
-15V: -15V1.TP -15V.TP C1N.2 C2N.2 C3N.2 C4N.2 C5N.2 C6N.2 C7N.2 C8N.2 C13.- CN3.- IC12*.4(P:V-) IC34*.4(P:V-) ; also sheet 1
GND: C1N.1 C1P.2 C2N.1 C2P.2 C3N.1 C3P.2 C4N.1 C4P.2 C5N.1 C5P.2 C6N.1 C6P.2 C7N.1 C7P.2 C8N.1 C8P.2 C9P.2 C10P.2 C11P.2 C13.+ C14.2 C15.- C16.2 C18.- C21.- C22.2 CN3.+ CP3.- GND1.TP GND.TP IC9.8(GND) IC10.8(GND) IC11.8(GND) IC12.2(GND) IC13.2(GND) LED1.C ; also sheet 1,2
N$7: LED1.A RLD.2

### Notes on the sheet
- IC12* | IC34*
- PCB1 Sheet 3: Power-Supply

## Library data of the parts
+5V +12V +15V +15V1 -15V -15V1 CON1 CON2 E1-E11 GND GND1 IC6.6 Q1G = testpad:TP: Test pad
C1 C1N C1P C2 C2N C2P C3 C3N C3P C4N C4P C5N C5P C6N C6P C7N C7P C8N C8P C9 C9P C10 C10P C11 C11P C12 C14 C16 C22 CKM1-CKM4 CLN1-CLN4 = rcl:C-EU: CAPACITOR, European symbol; SPICEPREFIX: C
C4-C8 C13 C15 C18 C21 CN3 CP3 = rcl:CPOL-EU: POLARIZED CAPACITOR, European symbol; SPICEPREFIX: C
CON3 = Wurth_Elektronik_Electromechanic_Wire_to_Board_Connectors_rev16a:61200821621: WR-BHD 2.54mm Male Box Header, 8 Pins=>Code : Con_WTB_BHD_2.54_Male_THT_WS_61200821621 Details see: http://katalog.we-online.de/en/em/612_0xx_216_21 Created 2014-06-04, Karrer Zheng 2014 (C) Würth Elektronik
D1-D3 = semicon-smd-ipc:D-: DIODE
DS1-DS14 DS17-DS24 = diode:DIODE-: DIODE
IC1-IC4 IC8 = linear:NE5534: LOW-NOISE OPERATIONAL AMPLIFIER Source: http://focus.ti.com/lit/ds/symlink/ne5534.pdf
IC5-IC7 = linear:LM318: OP AMP
IC9-IC11 = 74xx-eu:74*595: 8-bit SHIFT REGISTER, output latch
IC12 IC13 = linear:78*: Positive VOLTAGE REGULATOR Source: http://cache.national.com/ds/LM/LM78L05.pdf http://www.fairchildsemi.com/ds/LM/LM7805.pdf
IC12* IC34* = linear:OPA1013: OP AMP
K1-K14 K17-K24 = relay:G6K: Low Signal Relay oeiwcsnts1.omron.com/.. D20G6K0100.pdf; MF: OMRON COMPONENTS USA; MPN: G6K-2F-Y DC3; OC_FARNELL: 1690316; OC_NEWARK: 89C6451
LED1 = arduino:LED: LED
Q1 = transistor-small-signal:2N5638: N-CHANNEL FET
Q1* = transistor-small-signal:MMBFJ3*: N-Channel RF Amplifier Source: http://www.fairchildsemi.com/pf/J3/J310.html
Q2-Q4 = transistor:2N3904: NPN TRANSISTOR
QS1-QS14 QS17-QS24 = semicon-smd-ipc:NPN-TRANSISTOR_: NPN TRANSISTOR
R1-R4 R24 = rcl:R-TRIMM: Trimm resistor; SPICEMODEL: X; SPICEPREFIXL: POT
R5-R23 R25-R29 R31-R43 R205 R206 RE1-RE11 RF1-RF11 RKM4 RLD RLN4 = rcl:R-EU_: RESISTOR, European symbol; SPICEPREFIX: R
R30 = rcl:POTENTIOMETER_: Potentiometer; SPICEMODEL: POT; SPICEPREFIX: X
RS1-RS14 RS17-RS24 = rcl:R-EU_: RESISTOR, European symbol

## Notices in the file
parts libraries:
Wurth_Elektronik_Electromechanic_Wire_to: Copyright: Würth Elektronik
